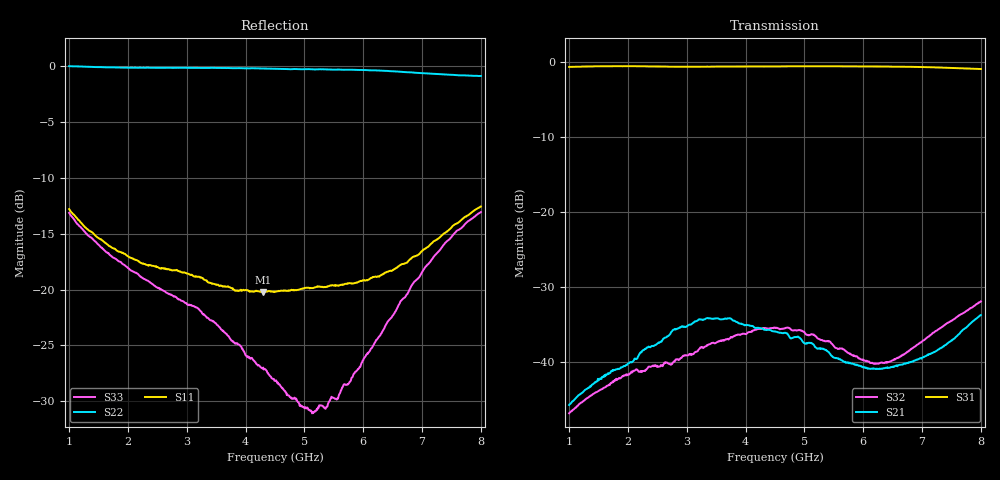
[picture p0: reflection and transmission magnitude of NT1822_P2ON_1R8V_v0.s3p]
! NT1822 PC-P2 ON state
! Port1:PC, Port2:P1, Port3:P2
! VDD=1.8V, VCTL=1.2V
# hz S ma R 50
! 3 Port Network Data from SP1.SP block
! freq  magS11  angS11  magS12  angS12  magS13  angS13
!  magS21  angS21
!  magS22  angS22  magS23  angS23
!  magS31  angS31  magS32  angS32
!  magS33  angS33
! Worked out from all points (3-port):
!   701 points, 1 GHz to 8 GHz, reference 50 ohm
!   strongest paths, dB at 1 GHz, 2.75 GHz, 4.5 GHz, 6.25 GHz, 8 GHz:
!     S31: -0.6, -0.6, -0.6, -0.6, -0.9
!     S21: -45.8, -35.9, -35.9, -41.0, -33.8
!     S32: -46.9, -40.3, -35.4, -40.3, -31.9
!   lowest |S11| = -20.2 dB at 4.3 GHz (marker M1), VSWR 1.22, Z = 54 - j9.36 ohm
!   |S11| at or under -10 dB: start of sweep to end of sweep
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1e9  0.2294 -76.4  0.005168 78.4  0.9312 1.6
     0.005139 78.7  1.002 -13.9  0.004522 73.1
     0.9308 1.4  0.004521 73.3  0.2206 -76.5
2.04e9  0.139 -77.3  0.009935 78.2  0.9417 -14.6
        0.009962 78.2  0.9862 -27.3  0.008371 68.5
        0.941 -14.8  0.008348 68.0  0.1223 -90.1
3.2e9  0.1144 -67.3  0.01916 64.3  0.9334 -27.1
       0.01913 64.4  0.9842 -41.4  0.01188 72.5
       0.9331 -27.4  0.01203 72.4  0.08183 -101.5
4.3e9  0.09736 -61.9  0.0166 42.2  0.9377 -38.2
       0.01654 42.6  0.9776 -56.1  0.01674 58.7
       0.937 -38.6  0.01681 58.1  0.04473 -122.3
4.5e9  0.09776 -63.0  0.01601 41.5  0.9384 -40.3
       0.01595 41.6  0.9748 -59.1  0.01681 54.7
       0.9377 -40.8  0.01692 54.3  0.03912 -124.5
5.12e9  0.1016 -71.2  0.01343 39.1  0.9395 -46.8
        0.01335 39.4  0.9702 -69.3  0.01517 45.9
        0.9393 -47.3  0.01529 45.3  0.02852 -119.1
5.36e9  0.1027 -76.9  0.01197 40.5  0.9398 -49.3
        0.01195 40.9  0.9694 -73.8  0.01366 45.5
        0.94 -49.8  0.01369 44.7  0.02924 -117.0
6.36e9  0.1183 -113.2  0.009057 74.6  0.9366 -60.1
        0.009044 74.2  0.9547 -94.5  0.009766 73.7
        0.9364 -60.6  0.009794 73.2  0.06721 -129.0
7.2e9  0.1647 -149.8  0.01159 104.8  0.925 -69.6
       0.0116 104.6  0.9249 -113.1  0.01571 102.5
       0.9252 -70.0  0.01563 102.2  0.1404 -137.4
8e9  0.2356 -173.7  0.02062 121.1  0.9012 -78.4
     0.02049 121.0  0.9054 -127.1  0.02527 109.1
     0.9012 -78.9  0.02529 108.3  0.2224 -141.7
